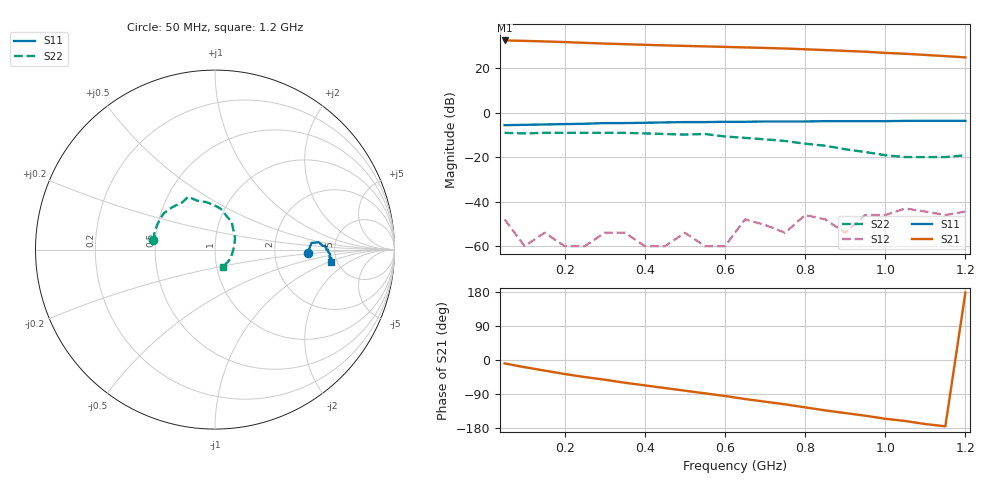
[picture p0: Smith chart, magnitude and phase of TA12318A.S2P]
!  ITA-12318  S-PARAMETERS
!  VCC - Vee =5 V  LAST UPDATED 07-22-92
# ghz s ma r 50
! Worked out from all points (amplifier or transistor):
!   24 points, 50 MHz to 1.2 GHz, reference 50 ohm
!   highest |S21| = 32.4 dB at 50 MHz (marker M1)
!   |S21| within 3 dB of that: start of sweep to 622.6 MHz
!   unconditionally stable (mu >= 1): start of sweep to end of sweep
!   at 250 MHz: K = 8.43, MAG = 33.4 dB, |S12| = -60.0 dB
!   at 650 MHz: K = 2.36, MAG = 32.1 dB, |S12| = -48.0 dB
!   at 1.2 GHz: K = 2.75, MAG = 27.4 dB, |S12| = -44.4 dB
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0.05  0.52 -2.0  41.51 -9.0  0.004 0.1  0.35 171.0
0.1  0.53 2.0  40.62 -19.0  0.001 -159.0  0.34 169.0
0.15  0.54 4.0  39.43 -28.0  0.002 -97.0  0.35 166.0
0.2  0.55 4.0  38.21 -37.0  0.001 86.0  0.35 162.0
0.25  0.56 4.0  36.65 -45.0  0.001 29.0  0.35 157.0
0.3  0.58 4.0  35.31 -52.0  0.002 48.0  0.35 151.0
0.35  0.58 4.0  34.26 -60.0  0.002 43.0  0.35 145.0
0.4  0.59 3.0  33.17 -67.0  0.001 95.0  0.34 138.0
0.45  0.6 2.0  32.16 -74.0  0.001 -96.0  0.33 132.0
0.5  0.61 2.0  31.31 -81.0  0.002 164.0  0.32 125.0
0.55  0.61 2.0  30.57 -88.0  0.001 -175.0  0.33 117.0
0.6  0.62 1.0  29.77 -95.0  0.001 -7.0  0.29 110.0
0.65  0.62 0.0  28.93 -103.0  0.004 -139.0  0.27 101.0
0.75  0.63 -1.0  27.36 -117.0  0.002 41.0  0.23 82.0
0.8  0.63 -1.0  26.3 -125.0  0.005 136.0  0.2 72.0
0.85  0.64 -2.0  25.26 -133.0  0.004 164.0  0.18 59.0
0.9  0.64 -3.0  24.21 -140.0  0.002 179.0  0.15 47.0
0.95  0.64 -3.0  23.2 -147.0  0.005 161.0  0.13 31.0
1  0.64 -4.0  21.81 -155.0  0.005 -178.0  0.11 12.0
1.05  0.65 -4.0  20.85 -161.0  0.007 125.0  0.1 -6.0
1.1  0.65 -5.0  19.64 -169.0  0.006 157.0  0.1 -32.0
1.2  0.65 -6.0  17.3 178.0  0.006 153.0  0.11 -65.0
